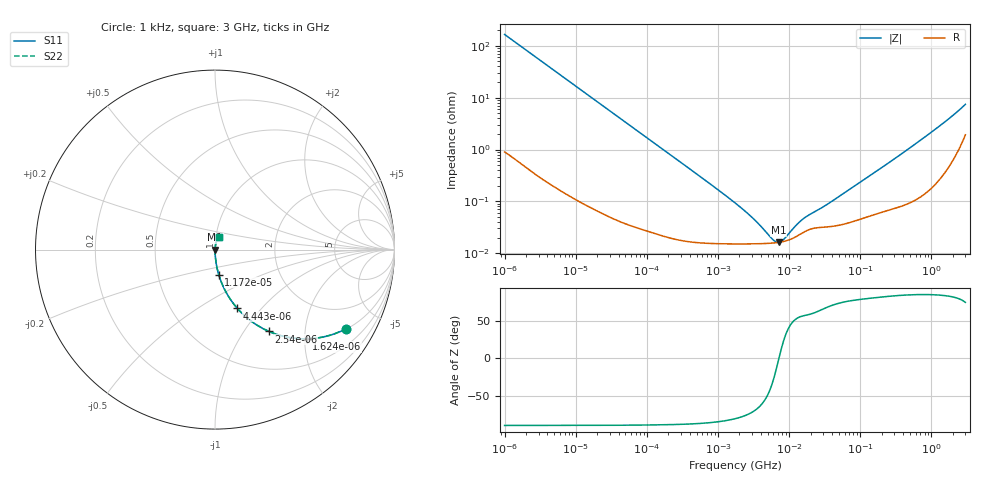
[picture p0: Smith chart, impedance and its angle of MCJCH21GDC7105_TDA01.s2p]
! MCJCH21GDC7105_TDA01  S-PARAMETER MODEL  ( Standard Model )
! Model Generated by TAIYO YUDEN Corporation (http://www.ty-top.com)
! Version 1.0
! TAIYO YUDEN Control No. 220601
! Copyright(c) 2018 TAIYO YUDEN CO.,LTD. All Rights Reserved.
! Product Description (link to TY-COMPAS)
! https://ds.yuden.co.jp/TYCOMPAS/or/detail?pn=MCJCH21GDC7105KTDA01&u=M
! Products Name : Multilayer Ceramic Capacitors
! Characteristics :
!  Capacitance : 1 [uF] , Rated Voltage : 100 [V] , TCC : X7S
!  Case Size : 2.0 x 1.25 / 0.079 x 0.049 [mm/inch] , Thickness : 1.25 / 0.049 [mm/inch]
!  (Conditions: Temperature = 25 [degC] , DC Bias Voltage = 0 [V])
! External Node Assignments :
!  1  o---| |---o  2
! GND o---------o GND
! Frequency Range : 1kHz  -  3GHz  [ 401 STEP ]
# MHZ S RI R 50
! Freq[MHz].  S11 Real  S11 Imag  S21 Real  S21 Imag  S12 Real  S12 Imag  S22 Real  S22 Imag
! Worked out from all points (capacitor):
!   401 points, 1 kHz to 3 GHz, reference 50 ohm
!   read as one part in series: C = 958 nF near 1.077 kHz
!   lowest |Z| = 16.2 mohm at 7.143 MHz (marker M1)
!   series resonance near 7.172 MHz, so ESL is about 510 pH
!   S11 on the Smith chart (normalised r, x): 1 kHz: 1.02, -3.32; 1.624 kHz: 1.01, -2.05; 2.54 kHz: 1.01, -1.31; 4.443 kHz: 1.00, -0.75; 11.71 kHz: 1.00, -0.29; 3 GHz: 1.04, +0.14
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0.001  0.7323 -0.4401  0.2677 0.4401  0.2677 0.4401  0.7323 -0.4401
0.001624  0.5116 -0.4972  0.4884 0.4972  0.4884 0.4972  0.5116 -0.4972
0.00254  0.3014 -0.4562  0.6986 0.4562  0.6986 0.4562  0.3014 -0.4562
0.003297  0.2046 -0.4007  0.7954 0.4007  0.7954 0.4007  0.2046 -0.4007
0.004443  0.1248 -0.3277  0.8752 0.3277  0.8752 0.3277  0.1248 -0.3277
0.006696  0.0598 -0.2341  0.9402 0.2341  0.9402 0.2341  0.0598 -0.2341
0.011715  0.0209 -0.1397  0.9791 0.1397  0.9791 0.1397  0.0209 -0.1397
0.01216  0.0195 -0.1348  0.9805 0.1348  0.9805 0.1348  0.0195 -0.1348
0.033275  0.003 -0.0503  0.997 0.0503  0.997 0.0503  0.003 -0.0503
0.147855  0.000357 -0.0114  0.9996 0.0114  0.9996 0.0114  0.000357 -0.0114
1.732051  0.000152 -0.000925  0.9998 0.000925  0.9998 0.000925  0.000152 -0.000925
3.264662  0.000152 -0.000414  0.9998 0.000414  0.9998 0.000414  0.000152 -0.000414
5.928204  0.000157 -9.18e-05  0.9998 9.18e-05  0.9998 9.18e-05  0.000157 -9.18e-05
6.629817  0.00016 -3.78e-05  0.9998 3.78e-05  0.9998 3.78e-05  0.00016 -3.78e-05
7.143107  0.000162 -1.94e-06  0.9998 1.94e-06  0.9998 1.94e-06  0.000162 -1.94e-06
8.606987  0.00017 8.83e-05  0.9998 -8.83e-05  0.9998 -8.83e-05  0.00017 8.83e-05
14.50609  0.000235 0.000348  0.9998 -0.000348  0.9998 -0.000348  0.000235 0.000348
21.06097  0.000298 0.000514  0.9997 -0.000514  0.9997 -0.000514  0.000298 0.000514
38.244  0.000327 0.00091  0.9997 -0.00091  0.9997 -0.00091  0.000327 0.00091
256.0921  0.00071 0.00561  0.9993 -0.00561  0.9993 -0.00561  0.00071 0.00561
1056.143  0.00244 0.0228  0.9976 -0.0228  0.9976 -0.0228  0.00244 0.0228
3000  0.0238 0.0689  0.9762 -0.0689  0.9762 -0.0689  0.0238 0.0689
